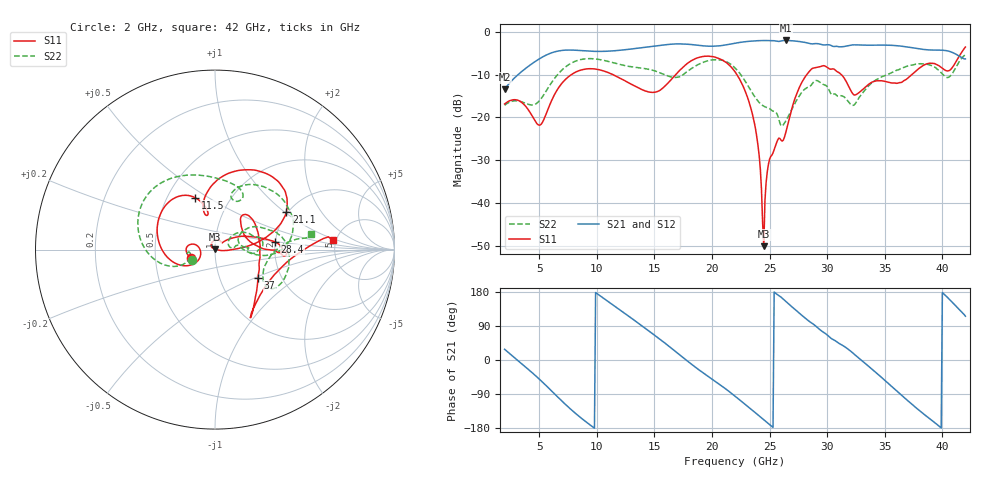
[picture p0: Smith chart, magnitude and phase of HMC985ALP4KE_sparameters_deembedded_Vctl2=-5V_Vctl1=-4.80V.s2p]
!s2p File: Measurements: S11, S21, S12, S22
# GHz S dB R 50.0
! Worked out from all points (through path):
!   401 points, 2 GHz to 42 GHz, reference 50 ohm
!   highest |S21| = -2.06 dB at 26.4 GHz (marker M1); lowest = -13.4 dB at 2 GHz (marker M2)
!   lowest |S11| = -50.0 dB at 24.5 GHz (marker M3), VSWR 1.01, Z = 49.8 + j0.265 ohm
!   |S11| at or under -10 dB: start of sweep to 7.809 GHz; 22.16 GHz to 28.24 GHz (6.081 GHz wide, 24.1 % of centre); 31.22 GHz to 37.36 GHz (6.144 GHz wide, 17.9 % of centre)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
!   |S22| runs from -22.0 to -5.4 dB; largest |S21 - S12| = 0.0011
!   S11 on the Smith chart (normalised r, x): 2 GHz: 0.76, -0.07; 11.5 GHz: 0.68, +0.44; 21.1 GHz: 1.96, +1.02; 28.4 GHz: 1.99, +0.19; 37 GHz: 1.52, -0.52; 42 GHz: 4.72, +0.86
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2  -16.88 -161.7  -13.43 28.3  -13.44 28.3  -17.18 -155.6
5  -21.80 -172.3  -6.37 -50.1  -6.38 -50.1  -16.18 -159.7
6.3  -14.84 -150.2  -4.76 -88.3  -4.76 -88.3  -11.03 -161.5
8.7  -8.91 150.4  -4.44 -154.5  -4.44 -154.5  -6.47 151.4
11.5  -10.16 111.1  -4.47 143.2  -4.47 143.2  -7.31 105.2
13.6  -13.11 101.2  -3.86 97.3  -3.86 97.3  -8.41 75.8
15.4  -13.82 105.8  -3.26 56.6  -3.26 56.6  -9.50 62.2
17.9  -7.34 80.4  -2.95 -3.4  -2.94 -3.3  -9.20 72.2
21.1  -6.96 27.7  -3.15 -74.2  -3.15 -74.2  -6.87 16.3
22  -9.35 17.2  -2.71 -95.4  -2.71 -95.3  -8.45 0.8
23.6  -20.25 0.0  -2.18 -135.0  -2.18 -135.0  -14.71 -4.2
24.5  -50.00 122.6  -2.08 -157.7  -2.08 -157.6  -17.38 8.1
25  -29.75 133.4  -2.11 -170.4  -2.11 -170.4  -17.95 10.9
26.4  -23.61 42.0  -2.06 154.9  -2.06 154.9  -20.86 33.2
28.4  -9.44 7.3  -2.72 103.0  -2.72 103.0  -12.88 18.7
28.7  -8.61 2.3  -2.86 96.7  -2.86 96.8  -12.19 16.7
30.7  -8.96 -2.8  -3.45 50.9  -3.45 50.9  -14.55 2.6
32.5  -14.70 31.9  -3.09 11.2  -3.09 11.3  -16.56 27.8
35.4  -11.82 19.4  -3.17 -64.3  -3.17 -64.2  -9.82 19.6
37  -10.84 -33.2  -3.60 -107.4  -3.60 -107.3  -8.03 5.3
39.8  -8.13 -57.0  -4.31 -176.8  -4.31 -176.7  -9.30 -35.2
42  -3.61 4.5  -6.36 115.6  -6.36 115.6  -5.36 9.0
